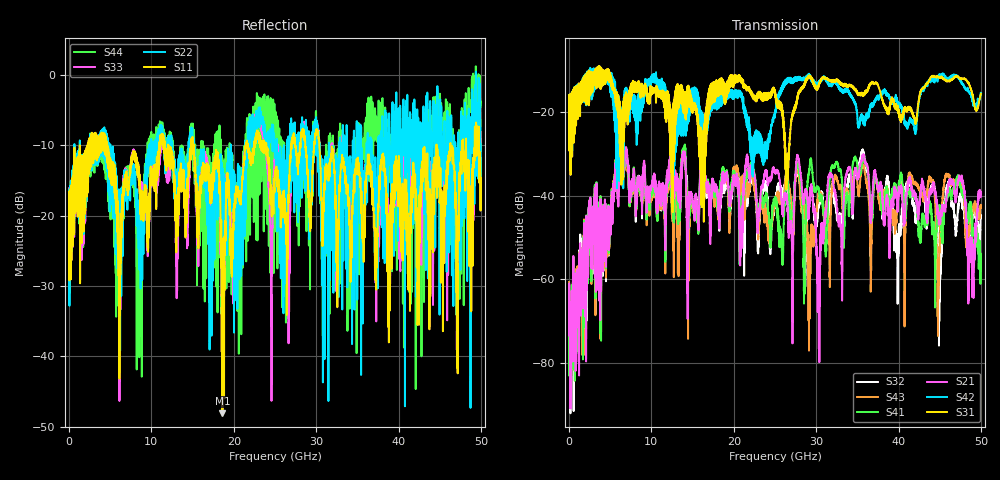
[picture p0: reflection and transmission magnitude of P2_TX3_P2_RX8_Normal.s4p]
!Keysight Technologies,N5225B,MY57041031,A.13.20.10
!Date: Friday, May 31, 2019 11:39:24
!Correction: S11(Full 4 Port(1,2,3,4))
!S12(Full 4 Port(1,2,3,4))
!S13(Full 4 Port(1,2,3,4))
!S14(Full 4 Port(1,2,3,4))
!S21(Full 4 Port(1,2,3,4))
!S22(Full 4 Port(1,2,3,4))
!S23(Full 4 Port(1,2,3,4))
!S24(Full 4 Port(1,2,3,4))
!S31(Full 4 Port(1,2,3,4))
!S32(Full 4 Port(1,2,3,4))
!S33(Full 4 Port(1,2,3,4))
!S34(Full 4 Port(1,2,3,4))
!S41(Full 4 Port(1,2,3,4))
!S42(Full 4 Port(1,2,3,4))
!S43(Full 4 Port(1,2,3,4))
!S44(Full 4 Port(1,2,3,4))
!S4P File: Measurements: <S11,S12,S13,S14>,
!<S21,S22,S23,S24>,
!<S31,S32,S33,S34>,
!<S41,S42,S43,S44>:
# Hz S  dB  R 50.0
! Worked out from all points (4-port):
!   5000 points, 10 MHz to 50 GHz, reference 50 ohm
!   strongest paths, dB at 10 MHz, 12.51 GHz, 25.01 GHz, 37.51 GHz, 50 GHz:
!     S31: -19.5, -42.6, -16.1, -13.6, -15.6
!     S42: -19.6, -21.5, -19.9, -16.3, -15.4
!     S21: -70.0, -37.2, -34.4, -38.5, -39.5
!     S41: -64.5, -40.0, -40.5, -37.6, -57.0
!     S43: -60.6, -40.7, -40.9, -39.0, -42.4
!     S32: -61.8, -38.1, -40.8, -37.9, -44.7
!   lowest |S11| = -48.1 dB at 18.62 GHz (marker M1), VSWR 1.01, Z = 49.8 - j0.316 ohm
!   |S11| at or under -10 dB: 4.63 GHz to 10.95 GHz (6.317 GHz wide, 81.1 % of centre); 15.14 GHz to 21.46 GHz (6.324 GHz wide, 34.6 % of centre); 30.38 GHz to 44.61 GHz (14.23 GHz wide, 37.9 % of centre)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
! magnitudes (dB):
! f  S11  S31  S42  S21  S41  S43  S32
! 10 MHz  -19.5  -19.5  -19.6  -70.0  -64.5  -60.6  -61.8
! 6.35 GHz  -19.7  -28.2  -24.2  -31.8  -30.9  -30.1  -30.8
! 18.62 GHz  -48.1  -12.3  -17.0  -34.6  -33.4  -35.4  -36.6
! 27.81 GHz  -12.9  -16.0  -12.0  -30.7  -32.8  -34.0  -34.8
! 30.26 GHz  -8.8  -13.9  -13.2  -57.5  -37.9  -39.6  -42.8
! 35.66 GHz  -23.2  -16.1  -21.0  -30.3  -31.3  -32.8  -28.9
! 50 GHz  -15.7  -15.6  -15.4  -39.5  -57.0  -42.4  -44.7
